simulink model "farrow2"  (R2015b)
settings: Solver=FixedStepDiscrete  StartTime=0.0  StopTime=10.0  RelTol=1e-3
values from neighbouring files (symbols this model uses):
  del = 0.8    [farrow_1.m]    (also in farrow_2.m = 0.45; farrow_4.m = mod(m*L/M, 1))
  Ts = 1/fs    (= 5e-05)    [basisband_1.m]    (also in basisband_2.m = 5e-06; dezimier_1.m = 0.0005; dezimier_11.m = 0.0005; dezimier_2.m = 0.0005)

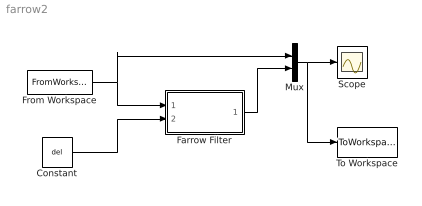
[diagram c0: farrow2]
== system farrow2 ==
  Constant : Constant  Value=del  SampleTime=Ts
  Farrow Filter : Subsystem  Tag=FilterWizardSubSystem
  From Workspace : FromWorkspace  VariableName=simin  SampleTime=Ts
  Mux : Mux  Inputs=2
  Scope : Scope
  To Workspace : ToWorkspace  VariableName=ysim  SaveFormat=Timeseries  SampleTime=-1
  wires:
  From Workspace/1 -> Farrow Filter/1(Input), Mux/1
  Constant/1 -> Farrow Filter/2(FracDelay)
  Farrow Filter/1(Output) -> Mux/2
  Mux/1 -> Scope/1, To Workspace/1

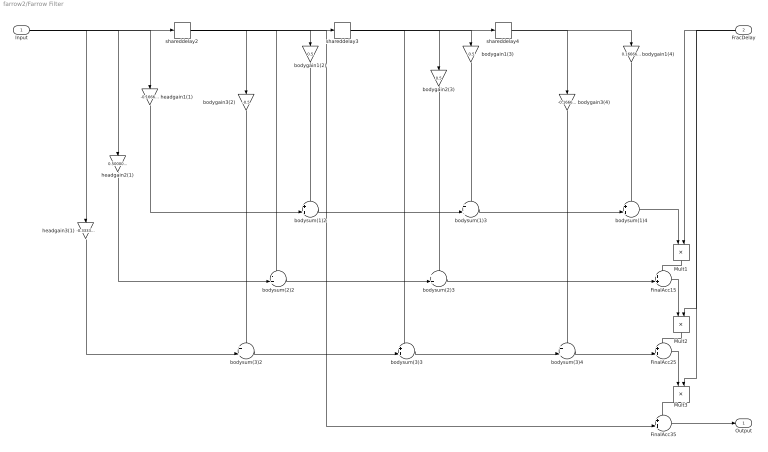
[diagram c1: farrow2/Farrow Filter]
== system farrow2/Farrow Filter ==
  Input : Inport
  FracDelay : Inport  Port=2
  FinalAcc15 : Sum  Inputs=++|  RndMeth=Nearest
  FinalAcc25 : Sum  Inputs=++|  RndMeth=Nearest
  FinalAcc35 : Sum  Inputs=++|  RndMeth=Nearest
  Mult1 : Product  RndMeth=Nearest
  Mult2 : Product  RndMeth=Nearest
  Mult3 : Product  RndMeth=Nearest
  bodygain1(2) : Gain  Gain=0.5  ParamDataTypeStr=double  RndMeth=Nearest
  bodygain1(3) : Gain  Gain=-0.5  ParamDataTypeStr=double  RndMeth=Nearest
  bodygain1(4) : Gain  Gain=0.166666666666666657  ParamDataTypeStr=double  RndMeth=Nearest
  bodygain2(3) : Gain  Gain=0.5  ParamDataTypeStr=double  RndMeth=Nearest
  bodygain3(2) : Gain  Gain=-0.5  ParamDataTypeStr=double  RndMeth=Nearest
  bodygain3(4) : Gain  Gain=-0.166666666666666741  ParamDataTypeStr=double  RndMeth=Nearest
  bodysum(1)2 : Sum  Inputs=++|  RndMeth=Nearest
  bodysum(1)3 : Sum  Inputs=++|  RndMeth=Nearest
  bodysum(1)4 : Sum  Inputs=++|  RndMeth=Nearest
  bodysum(2)2 : Sum  Inputs=-+|  RndMeth=Nearest
  bodysum(2)3 : Sum  Inputs=++|  RndMeth=Nearest
  bodysum(3)2 : Sum  Inputs=++|  RndMeth=Nearest
  bodysum(3)3 : Sum  Inputs=++|  RndMeth=Nearest
  bodysum(3)4 : Sum  Inputs=++|  RndMeth=Nearest
  headgain1(1) : Gain  Gain=-0.16666666666666663  ParamDataTypeStr=double  RndMeth=Nearest
  headgain2(1) : Gain  Gain=0.500000000000000111  ParamDataTypeStr=double  RndMeth=Nearest
  headgain3(1) : Gain  Gain=-0.333333333333333148  ParamDataTypeStr=double  RndMeth=Nearest
  shareddelay2 : Delay  DelayLength=1  InitialCondition=0  InputProcessing=Columns as channels (frame based)
  shareddelay3 : Delay  DelayLength=1  InitialCondition=0  InputProcessing=Columns as channels (frame based)
  shareddelay4 : Delay  DelayLength=1  InitialCondition=0  InputProcessing=Columns as channels (frame based)
  Output : Outport
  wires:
  headgain1(1)/1 -> bodysum(1)2/2
  headgain2(1)/1 -> bodysum(2)2/2
  headgain3(1)/1 -> bodysum(3)2/2
  Input/1 -> headgain1(1)/1, headgain2(1)/1, headgain3(1)/1, shareddelay2/1
  bodygain1(2)/1 -> bodysum(1)2/1
  bodygain3(2)/1 -> bodysum(3)2/1
  bodysum(1)2/1 -> bodysum(1)3/2
  bodysum(2)2/1 -> bodysum(2)3/2
  bodysum(3)2/1 -> bodysum(3)3/2
  shareddelay2/1 -> bodygain1(2)/1, bodysum(2)2/1, bodygain3(2)/1, FinalAcc35/2, shareddelay3/1
  bodygain1(3)/1 -> bodysum(1)3/1
  bodygain2(3)/1 -> bodysum(2)3/1
  bodysum(1)3/1 -> bodysum(1)4/2
  bodysum(2)3/1 -> FinalAcc15/2
  bodysum(3)3/1 -> bodysum(3)4/2
  shareddelay3/1 -> bodygain1(3)/1, bodygain2(3)/1, bodysum(3)3/1, shareddelay4/1
  bodygain1(4)/1 -> bodysum(1)4/1
  bodygain3(4)/1 -> bodysum(3)4/1
  bodysum(1)4/1 -> Mult1/1
  bodysum(3)4/1 -> FinalAcc25/2
  shareddelay4/1 -> bodygain1(4)/1, bodygain3(4)/1
  FracDelay/1 -> Mult1/2, Mult2/2, Mult3/2
  Mult1/1 -> FinalAcc15/1
  FinalAcc15/1 -> Mult2/1
  Mult2/1 -> FinalAcc25/1
  FinalAcc25/1 -> Mult3/1
  Mult3/1 -> FinalAcc35/1
  FinalAcc35/1 -> Output/1
